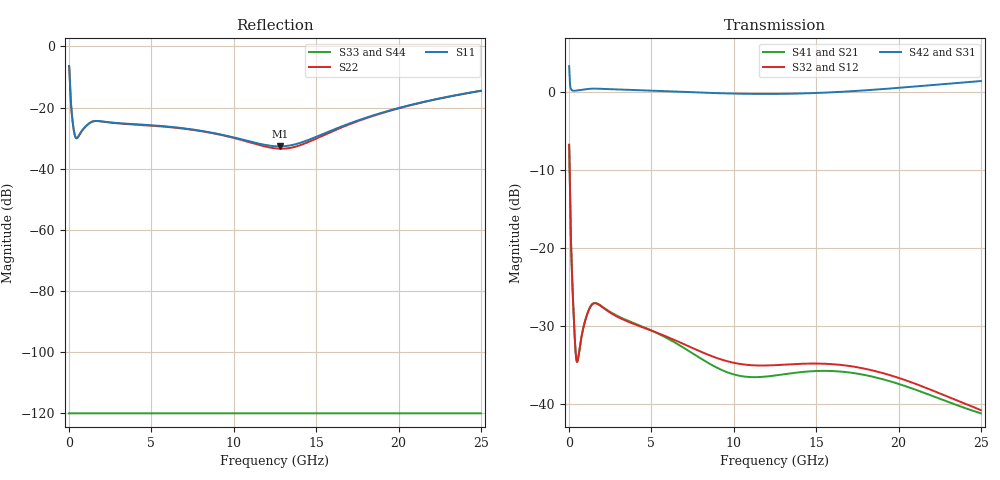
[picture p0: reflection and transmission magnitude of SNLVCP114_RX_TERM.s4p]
! Copyright 2008, Texas Instruments Incorporated. All rights reserved.
! Generated by program util_convert_RxTerm_to_s4p on 08-06-2012 14:24:05
!  1 ----xxxxxxxxxxxxxxxxxx---- 3
!  xxxxxxxxxxxxxxxxxx
!  (Input) xxxxxxxxxxxxxxxxxx  (Output)
!  xxxxxxxxxxxxxxxxxx
!  2 ----xxxxxxxxxxxxxxxxxx---- 4
! FREQ  S11  S12  S13  S14
!  S21  S22  S23  S24
!  S31  S32  S33  S34
!  S41  S42  S43  S44
!  DB  ANG  DB  ANG  DB  ANG  DB  ANG
# HZ S DB R 50.00
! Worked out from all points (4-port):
!   2501 points, 1 MHz to 25 GHz, reference 50 ohm
!   strongest paths, dB at 1 MHz, 6.251 GHz, 12.5 GHz, 18.75 GHz, 25 GHz:
!     S42: 3.4, 0.1, -0.2, 0.4, 1.5
!     S31: 3.4, 0.1, -0.2, 0.4, 1.5
!     S32: -6.7, -31.6, -35.0, -35.9, -40.8
!     S12: -6.7, -31.6, -35.0, -35.9, -40.8
!     S41: -6.7, -31.9, -36.3, -36.7, -41.2
!     S21: -6.7, -31.9, -36.3, -36.7, -41.2
!   lowest |S11| = -32.7 dB at 12.79 GHz (marker M1), VSWR 1.05, Z = 47.8 + j0.517 ohm
!   |S11| at or under -10 dB: 33 MHz to end of sweep
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1000000  -6.47 -2.8  -6.72 -1.0  -120.00 0.0  -120.00 0.0
         -6.72 -1.0  -6.47 -2.8  -120.00 0.0  -120.00 0.0
         3.37 -0.9  -6.72 -1.0  -120.00 0.0  -120.00 0.0
         -6.72 -1.0  3.37 -0.9  -120.00 0.0  -120.00 0.0
2.51e8  -26.16 -58.8  -27.32 -73.4  -120.00 0.0  -120.00 0.0
        -27.32 -73.3  -26.17 -58.8  -120.00 0.0  -120.00 0.0
        0.23 -2.3  -27.32 -73.4  -120.00 0.0  -120.00 0.0
        -27.32 -73.3  0.23 -2.3  -120.00 0.0  -120.00 0.0
5.01e8  -29.89 -16.2  -34.57 -22.5  -120.00 0.0  -120.00 0.0
        -34.54 -22.6  -29.91 -16.1  -120.00 0.0  -120.00 0.0
        0.26 -0.5  -34.57 -22.5  -120.00 0.0  -120.00 0.0
        -34.54 -22.6  0.26 -0.5  -120.00 0.0  -120.00 0.0
1.601e9  -24.38 -14.1  -27.06 -8.4  -120.00 0.0  -120.00 0.0
         -27.02 -8.8  -24.42 -13.9  -120.00 0.0  -120.00 0.0
         0.50 -0.8  -27.06 -8.4  -120.00 0.0  -120.00 0.0
         -27.02 -8.8  0.49 -0.8  -120.00 0.0  -120.00 0.0
9.541e9  -29.19 -119.9  -34.47 -36.1  -120.00 0.0  -120.00 0.0
         -35.87 -39.8  -29.33 -115.3  -120.00 0.0  -120.00 0.0
         -0.15 -1.8  -34.47 -36.1  -120.00 0.0  -120.00 0.0
         -35.87 -39.8  -0.12 -1.8  -120.00 0.0  -120.00 0.0
1.2791e10  -32.70 166.5  -34.98 -29.3  -120.00 0.0  -120.00 0.0
           -36.25 -26.1  -33.45 170.3  -120.00 0.0  -120.00 0.0
           -0.20 0.3  -34.98 -29.3  -120.00 0.0  -120.00 0.0
           -36.25 -26.1  -0.18 0.2  -120.00 0.0  -120.00 0.0
2.5001e10  -14.51 13.0  -40.78 -44.0  -120.00 0.0  -120.00 0.0
           -41.19 -34.8  -14.54 12.7  -120.00 0.0  -120.00 0.0
           1.47 2.1  -40.78 -44.0  -120.00 0.0  -120.00 0.0
           -41.19 -34.8  1.46 2.0  -120.00 0.0  -120.00 0.0
